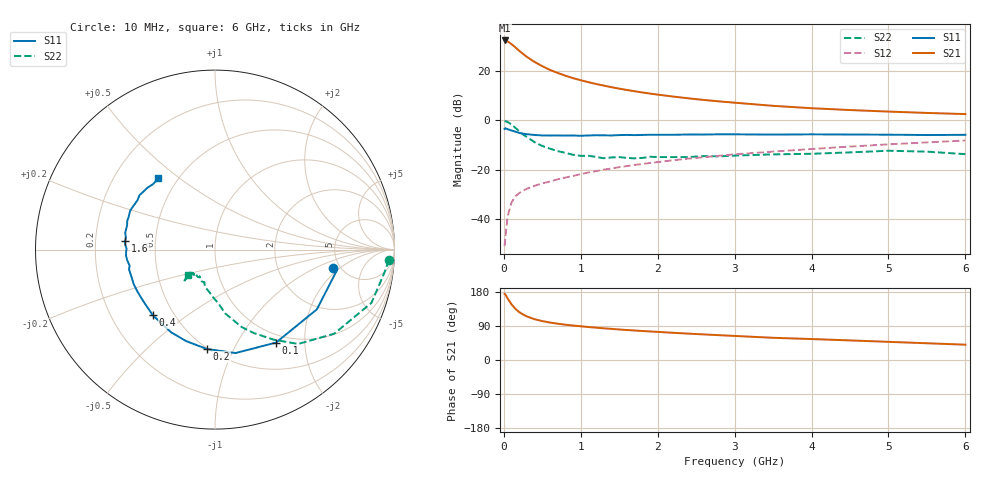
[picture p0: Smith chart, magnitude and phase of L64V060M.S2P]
!  INFINEON TECHNOLOGIES Small Signal Semiconductors
! BFR380L3 , Si-NPN RF-Transistor in TSLP-3-1
!  Vce=4 V,  Ic=60 mA
! Common Emitter S-Parameters:  07. March 2005
#  GHz  S  MA  R  50
! f  S11  S21  S12  S22
! GHz  Mag  Ang  Mag  Ang  Mag  Ang  Mag  Ang
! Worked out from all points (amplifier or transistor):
!   36 points, 10 MHz to 6 GHz, reference 50 ohm
!   highest |S21| = 32.1 dB at 10 MHz (marker M1)
!   |S21| within 3 dB of that: start of sweep to 157.8 MHz
!   unconditionally stable (mu >= 1): 1.586 GHz to 4.83 GHz
!   at 250 MHz: K = 0.46, MSG = 27.5 dB, |S12| = -28.4 dB
!   at 1.4 GHz: K = 0.99, MSG = 16.4 dB, |S12| = -19.5 dB
!   at 6 GHz: K = 0.97, MSG = 5.3 dB, |S12| = -8.2 dB
!   S11 on the Smith chart (normalised r, x): 10 MHz: 4.37, -1.60; 100 MHz: 0.88, -1.47; 200 MHz: 0.49, -0.79; 400 MHz: 0.38, -0.38; 1.6 GHz: 0.33, +0.04; 6 GHz: 0.39, +0.42
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0.01  0.6661 -8.8  40.32 174.5  0.0029 79.4  0.9704 -3.4
0.02  0.6883 -9.8  39.97 172.9  0.0044 86.4  0.9536 -7.5
0.05  0.658 -30.4  38.45 162.0  0.0118 79.7  0.9209 -18.8
0.1  0.6197 -56.7  33.99 146.9  0.022 67.4  0.8128 -35.2
0.15  0.5876 -78.8  29.26 135.0  0.0293 60.4  0.701 -48.6
0.2  0.5553 -94.8  24.98 126.4  0.034 56.9  0.6002 -56.8
0.25  0.5345 -107.6  21.61 120.1  0.038 54.9  0.5125 -65.1
0.3  0.5216 -118.0  18.79 114.9  0.0416 54.4  0.4572 -70.9
0.4  0.5039 -133.5  14.88 107.6  0.0477 54.4  0.3611 -80.8
0.5  0.4924 -143.7  12.22 102.7  0.0535 56.0  0.3023 -86.2
0.6  0.4915 -151.4  10.29 98.8  0.058 57.1  0.2667 -92.0
0.7  0.4921 -156.8  8.938 95.8  0.0645 59.3  0.2383 -97.7
0.9  0.4917 -167.0  7.021 90.9  0.0752 61.4  0.2008 -107.2
1.1  0.4924 -172.9  5.815 87.0  0.0885 63.3  0.1921 -112.6
1.3  0.4953 -178.9  4.965 83.5  0.1009 64.4  0.1714 -119.9
1.6  0.5048 174.5  4.054 79.1  0.1191 65.3  0.1737 -128.0
2.2  0.5078 164.8  2.99 71.8  0.1558 66.1  0.1804 -130.5
2.8  0.5192 156.0  2.39 65.5  0.1919 66.1  0.1867 -137.1
3.5  0.5121 147.5  1.944 58.6  0.2327 64.0  0.2047 -135.7
4.5  0.514 141.5  1.6 51.7  0.2941 62.3  0.2246 -135.2
5.5  0.5022 133.4  1.399 44.2  0.3569 58.6  0.2324 -134.6
6  0.5069 128.4  1.326 40.4  0.3894 56.4  0.2069 -136.4
